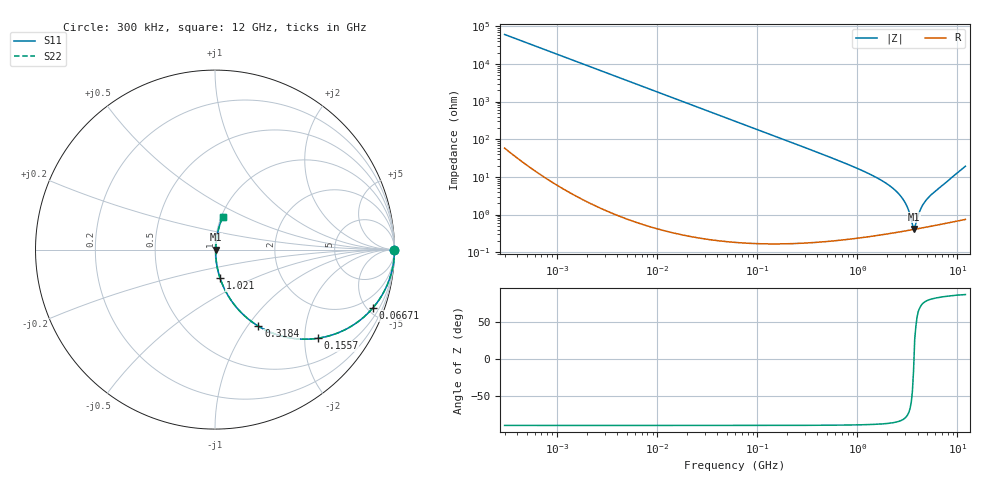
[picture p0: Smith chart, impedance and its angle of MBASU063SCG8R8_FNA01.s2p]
! MBASU063SCG8R8_FNA01  S-PARAMETER MODEL  ( General Type )
! Model Generated by TAIYO YUDEN Corporation (http://www.ty-top.com)
! Version 1.0
! TAIYO YUDEN Control No. 130801
! Copyright(c) 2013 TAIYO YUDEN CO.,LTD. All Rights Reserved.
! Product Description (link to TY-COMPAS)
! https://ds.yuden.co.jp/TYCOMPAS/or/detail?pn=MBASU063SCG8R8DFNA01&u=M
! Products Name : Multilayer Ceramic Capacitors
! Characteristics :
!  Capacitance : 8.8 pF , Rated Voltage : 50V , TCC : CG / C0G
!  Case Size : 0.6 x 0.3 / 0.024 x 0.012 [mm/inch] , Thickness : 0.3 / 0.012 [mm/inch]
!  (Conditions: Temperature = 25 degC , DC Bias Current/Voltage = 0A / 0V)
! External Node Assignments :
!  1  o---| |---o  2
! GND o---------o GND
! Frequency Range : 0.3MHz  -  12000MHz  [ 401 STEP ]
# MHz S RI R 50
! Freq[MHz].  S11 Real  S11 Imag  S21 Real  S21 Imag  S12 Real  S12 Imag  S22 Real  S22 Imag
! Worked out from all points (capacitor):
!   401 points, 300 kHz to 12 GHz, reference 50 ohm
!   read as one part in series: C = 8.79 pF near 316.3 kHz
!   lowest |Z| = 417 mohm at 3.643 GHz (marker M1)
!   series resonance near 3.678 GHz, so ESL is about 210 pH
!   S11 on the Smith chart (normalised r, x): 300 kHz: open; 66.71 MHz: 1.00, -5.43; 155.7 MHz: 1.00, -2.32; 318.4 MHz: 1.00, -1.13; 1.021 GHz: 1.00, -0.33; 12 GHz: 1.01, +0.38
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0.3  1 -0.00166  4.34e-06 0.00166  4.34e-06 0.00166  1 -0.00166
1.769972  0.9999 -0.00978  9.8e-05 0.00978  9.8e-05 0.00978  0.9999 -0.00978
10.44266  0.9967 -0.0575  0.00333 0.0575  0.00333 0.0575  0.9967 -0.0575
26.39317  0.9791 -0.1428  0.0209 0.1428  0.0209 0.1428  0.9791 -0.1428
60  0.9008 -0.2986  0.0992 0.2986  0.0992 0.2986  0.9008 -0.2986
66.70707  0.8802 -0.3244  0.1198 0.3244  0.1198 0.3244  0.8802 -0.3244
155.7172  0.5738 -0.4938  0.4262 0.4938  0.4262 0.4938  0.5738 -0.4938
318.4019  0.2422 -0.4269  0.7578 0.4269  0.7578 0.4269  0.2422 -0.4269
353.9943  0.2051 -0.402  0.7949 0.402  0.7949 0.402  0.2051 -0.402
570.2811  0.0891 -0.2817  0.9109 0.2817  0.9109 0.2817  0.0891 -0.2817
1021.415  0.0283 -0.1586  0.9717 0.1586  0.9717 0.1586  0.0283 -0.1586
2088.533  0.00653 -0.0583  0.9935 0.0583  0.9935 0.0583  0.00653 -0.0583
2581.562  0.00467 -0.0355  0.9953 0.0355  0.9953 0.0355  0.00467 -0.0355
2947.191  0.0041 -0.022  0.9959 0.022  0.9959 0.022  0.0041 -0.022
3190.978  0.00395 -0.0141  0.9961 0.0141  0.9961 0.0141  0.00395 -0.0141
3547.679  0.00395 -0.00375  0.996 0.00375  0.996 0.00375  0.00395 -0.00375
3642.919  0.00399 -0.00113  0.996 0.00113  0.996 0.00113  0.00399 -0.00113
3841.137  0.00411 0.00398  0.9959 -0.00398  0.9959 -0.00398  0.00411 0.00398
4158.869  0.00437 0.0107  0.9956 -0.0107  0.9956 -0.0107  0.00437 0.0107
4502.883  0.00472 0.0173  0.9953 -0.0173  0.9953 -0.0173  0.00472 0.0173
5140.631  0.00549 0.0277  0.9945 -0.0277  0.9945 -0.0277  0.00549 0.0277
12000  0.0418 0.1817  0.9582 -0.1817  0.9582 -0.1817  0.0418 0.1817
